(* 	
	Program Name: 	ACS_MOVE_VELOCITY_ROTARY_REVERSE
	Purpose:		Copy Velocity Move Profile to ACS Drive Output Registers
	When Executed:	Primes Output Registers for an Velocity Move in the reverse direction to be executed upon Start Motion command
	Notes:			Velocity Feed Forward must be set to 100% for this to properly run at defined velocity (In TMI tuning filter)
*)
PROGRAM ACS_MOVE_VELOCITY_ROTARY_REVERSE
VAR_IN_OUT
	Axis:ACS_DRIVE_TYPE;
END_VAR

VAR_INPUT
	// Final Velocity in rotary units
	ProfileVelocity		:REAL;
	// Acceleration in rotary units
	ProfileAcceleration	:REAL;
	//Deceleration in rotary units
	ProfileDeceleration	:REAL;
	// Force as % Peak motor current
	ProfileForce		:REAL;
END_VAR

VAR
	_moveType:UDINT := ACS_MOTION_TYPES.ROTARY_VELOCITY_REV;
	// Target Index
	_moveSelect:USINT := 0;
END_VAR

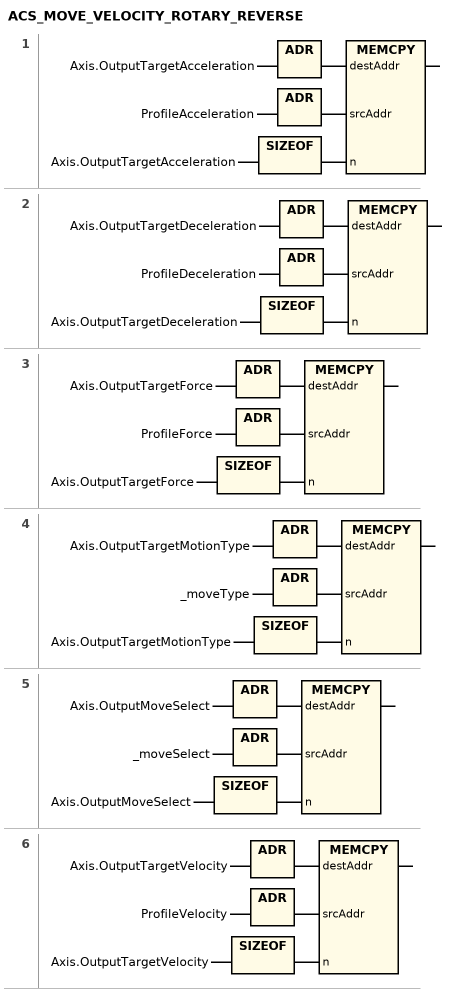
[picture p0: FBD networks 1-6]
// NETWORK 1
MEMCPY(destAddr := ADR(Axis.OutputTargetAcceleration), srcAddr := ADR(ProfileAcceleration), n := SIZEOF(Axis.OutputTargetAcceleration));

// NETWORK 2
MEMCPY(destAddr := ADR(Axis.OutputTargetDeceleration), srcAddr := ADR(ProfileDeceleration), n := SIZEOF(Axis.OutputTargetDeceleration));

// NETWORK 3
MEMCPY(destAddr := ADR(Axis.OutputTargetForce), srcAddr := ADR(ProfileForce), n := SIZEOF(Axis.OutputTargetForce));

// NETWORK 4
MEMCPY(destAddr := ADR(Axis.OutputTargetMotionType), srcAddr := ADR(_moveType), n := SIZEOF(Axis.OutputTargetMotionType));

// NETWORK 5
MEMCPY(destAddr := ADR(Axis.OutputMoveSelect), srcAddr := ADR(_moveSelect), n := SIZEOF(Axis.OutputMoveSelect));

// NETWORK 6
MEMCPY(destAddr := ADR(Axis.OutputTargetVelocity), srcAddr := ADR(ProfileVelocity), n := SIZEOF(Axis.OutputTargetVelocity));

END_PROGRAM
